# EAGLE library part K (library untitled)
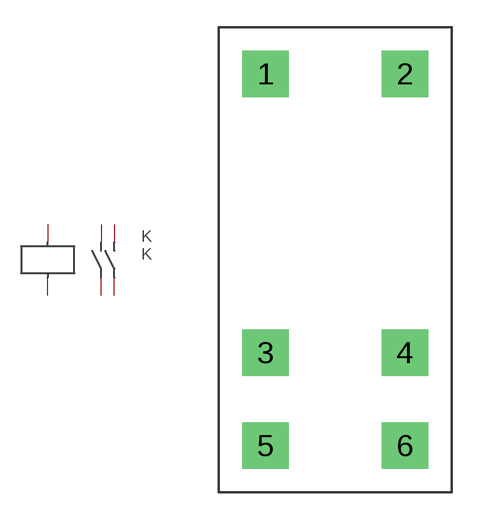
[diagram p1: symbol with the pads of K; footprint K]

Designator prefix K

## K  [K]
1  1
2  2
3  3
4  5
5  4
6  6

## Footprint K (pad centres in mm)
drill 0.5 pad 2.54 square: 1 0,16.51; 2 7.62,16.51; 3 0,1.27; 4 7.62,1.27; 5 0,-3.81; 6 7.62,-3.81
